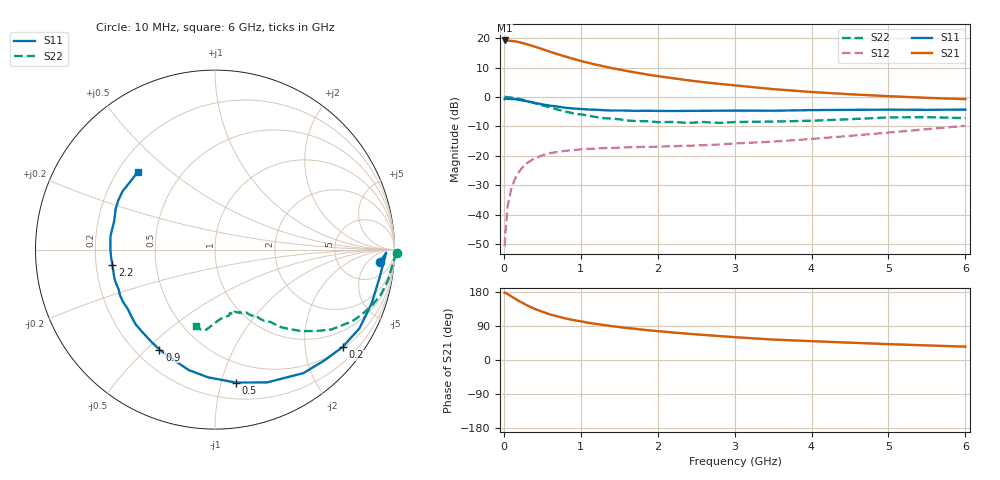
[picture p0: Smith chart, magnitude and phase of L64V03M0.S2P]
!  INFINEON TECHNOLOGIES Small Signal Semiconductors
! BFR380L3 , Si-NPN RF-Transistor in TSLP-3-1
!  Vce=4 V,  Ic=3 mA
! Common Emitter S-Parameters:  07. March 2005
#  GHz  S  MA  R  50
! f  S11  S21  S12  S22
! GHz  Mag  Ang  Mag  Ang  Mag  Ang  Mag  Ang
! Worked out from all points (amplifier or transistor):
!   36 points, 10 MHz to 6 GHz, reference 50 ohm
!   highest |S21| = 19.2 dB at 10 MHz (marker M1)
!   |S21| within 3 dB of that: start of sweep to 505.2 MHz
!   unconditionally stable (mu >= 1): 2.724 GHz to 4.615 GHz
!   at 250 MHz: K = 0.11, MSG = 21.0 dB, |S12| = -23.7 dB
!   at 1.4 GHz: K = 0.63, MSG = 13.6 dB, |S12| = -17.4 dB
!   at 6 GHz: K = 0.90, MSG = 4.5 dB, |S12| = -9.8 dB
!   S11 on the Smith chart (normalised r, x): 10 MHz: 13, -12; 200 MHz: 0.53, -2.87; 500 MHz: 0.33, -1.11; 900 MHz: 0.29, -0.55; 2.2 GHz: 0.27, -0.07; 6 GHz: 0.28, +0.39
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0.01  0.9217 -4.3  9.157 177.0  0.0029 90.0  1.015 -1.1
0.02  0.9543 -1.0  9.11 177.8  0.0049 87.5  1.005 -2.2
0.05  0.9298 -9.7  9.113 173.7  0.0142 85.6  0.992 -5.1
0.1  0.9231 -18.8  8.977 167.6  0.0285 81.1  0.978 -10.2
0.15  0.9167 -28.6  8.816 161.3  0.0418 74.9  0.9574 -15.2
0.2  0.8942 -37.4  8.546 155.2  0.0539 71.4  0.9298 -19.4
0.3  0.8463 -54.4  7.888 144.4  0.0747 61.9  0.8623 -27.6
0.4  0.7948 -68.6  7.206 135.0  0.0908 55.2  0.7878 -34.4
0.5  0.7494 -81.2  6.517 127.3  0.1015 50.0  0.7213 -39.0
0.6  0.7126 -93.1  5.885 120.3  0.1108 45.9  0.663 -43.2
0.7  0.6868 -102.3  5.338 114.9  0.1166 42.9  0.612 -46.5
0.8  0.6558 -110.8  4.873 109.8  0.1216 40.3  0.5673 -49.6
0.9  0.6375 -119.1  4.459 105.5  0.1253 38.4  0.5276 -51.5
1.1  0.613 -131.0  3.808 98.2  0.1311 36.4  0.4825 -55.4
1.3  0.5957 -141.7  3.329 92.3  0.1353 35.5  0.4351 -58.0
1.6  0.5872 -154.5  2.77 84.5  0.1391 35.5  0.3984 -63.0
2.2  0.578 -171.4  2.084 72.5  0.1459 39.3  0.3763 -69.2
2.8  0.5844 175.5  1.673 63.2  0.1557 45.3  0.3623 -76.7
3.5  0.5842 163.8  1.361 53.9  0.1741 51.5  0.3822 -83.6
4.5  0.6046 153.2  1.113 45.7  0.2182 60.2  0.4189 -91.7
5.5  0.605 141.6  0.968 38.5  0.2833 63.5  0.454 -99.8
6  0.6103 134.9  0.919 35.3  0.3236 63.3  0.437 -103.8
